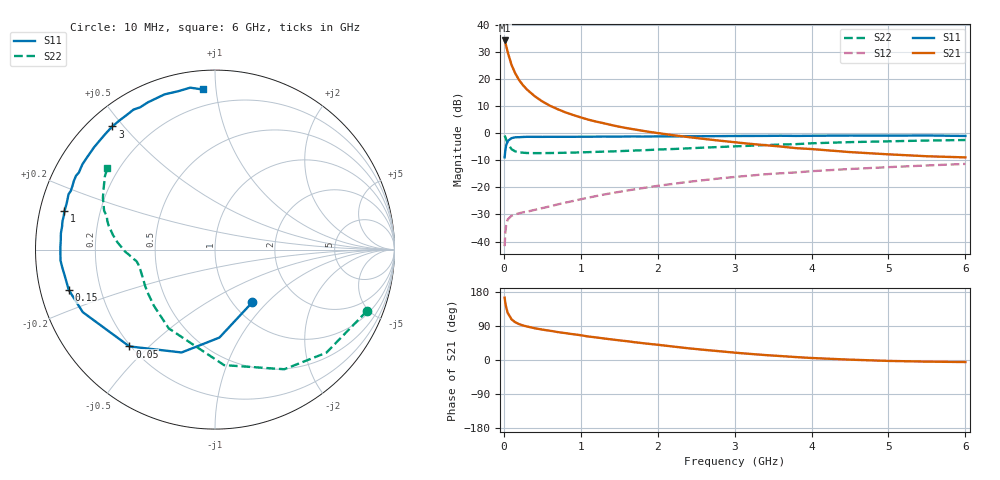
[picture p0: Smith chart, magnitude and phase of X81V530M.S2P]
! SIEMENS Small Signal Semiconductors
! BFP136W
! Si NPN RF Bipolar Junction Transistor in SOT343
! VCE = 1.5 V  IC = 30 mA
! Common Emitter S-Parameters:  September  1994
# GHz  S  MA  R  50
!  f  S11  S21  S12  S22
! GHz  MAG  ANG  MAG  ANG  MAG  ANG  MAG  ANG
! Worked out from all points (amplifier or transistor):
!   40 points, 10 MHz to 6 GHz, reference 50 ohm
!   highest |S21| = 34.3 dB at 10 MHz (marker M1)
!   |S21| within 3 dB of that: start of sweep to 38.98 MHz
!   unconditionally stable (mu >= 1): 707.3 MHz to 2.885 GHz
!   at 200 MHz: K = 0.43, MSG = 24.6 dB, |S12| = -29.6 dB
!   at 1.5 GHz: K = 1.15, MAG = 9.7 dB, |S12| = -21.6 dB
!   at 6 GHz: K = 1.00, MSG = 1.2 dB, |S12| = -11.3 dB
!   S11 on the Smith chart (normalised r, x): 10 MHz: 1.22, -0.82; 50 MHz: 0.19, -0.44; 150 MHz: 0.09, -0.13; 1 GHz: 0.07, +0.12; 3 GHz: 0.07, +0.47; 6 GHz: 0.10, +0.92
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0.01  0.3597 -54.7  52.17 164.4  0.0082 72.8  0.9132 -22.0
0.02  0.4907 -87.1  46.99 150.4  0.0149 61.7  0.8455 -42.8
0.03  0.6027 -108.0  41.79 139.5  0.0199 52.6  0.7704 -59.9
0.05  0.7201 -131.5  31.73 124.4  0.0256 39.1  0.6457 -85.5
0.1  0.8151 -154.7  18.42 107.3  0.03 28.0  0.5091 -120.4
0.15  0.8453 -164.6  12.69 99.3  0.0318 27.5  0.4626 -137.3
0.2  0.8492 -169.8  9.567 94.6  0.0333 27.1  0.4459 -146.8
0.25  0.8572 -173.5  7.732 91.1  0.0347 28.7  0.4385 -152.9
0.3  0.8629 -176.0  6.47 88.5  0.0355 30.3  0.4329 -157.0
0.4  0.8617 179.4  4.872 83.9  0.0384 34.1  0.4307 -162.2
0.5  0.8609 176.3  3.888 80.2  0.0415 37.7  0.4309 -165.5
0.6  0.8634 174.0  3.241 77.2  0.0447 40.6  0.4325 -167.5
0.8  0.8643 169.5  2.447 70.9  0.0523 46.1  0.4377 -170.1
1  0.8655 165.7  1.973 65.4  0.0604 49.3  0.445 -172.0
1.1  0.8655 162.9  1.787 61.9  0.0647 50.4  0.4492 -172.6
1.5  0.8695 156.1  1.325 51.9  0.0828 53.5  0.4684 -175.1
2.2  0.879 143.7  0.924 35.5  0.1164 52.4  0.5132 179.5
3  0.8934 129.8  0.685 19.4  0.1561 47.2  0.5748 171.8
3.2  0.8951 126.4  0.64 16.1  0.1652 45.6  0.5894 169.6
4.5  0.9095 108.0  0.45 0.9  0.2191 34.0  0.6881 155.2
5.5  0.9127 98.7  0.377 -4.3  0.2547 25.8  0.7363 146.5
6  0.8947 94.4  0.359 -5.4  0.2719 21.4  0.7528 142.8
